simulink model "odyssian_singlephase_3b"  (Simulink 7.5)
settings: Solver=ode23t  StartTime=0.0  StopTime=10  RelTol=1e-6
undefined symbols (not defined in the file or in its folder): dfilt, DiscIntNeverNeededParam
libraries: powerlib x36, powerlib_extras x15, simulink x12, dsparch4 x2

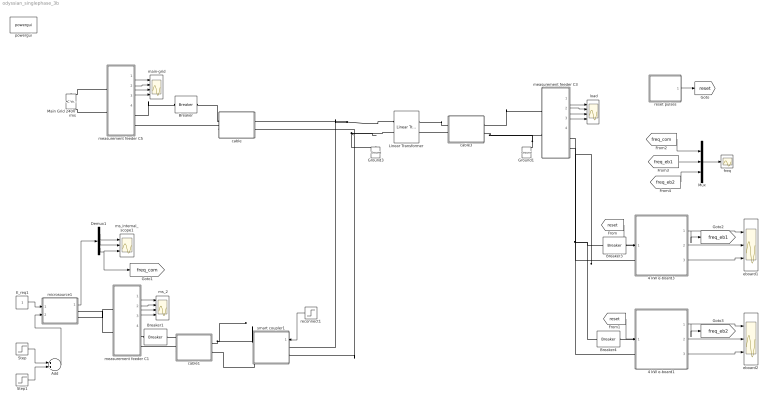
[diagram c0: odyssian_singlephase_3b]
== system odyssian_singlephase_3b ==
  " load" : Scope  NumInputPorts=4
  " main-grid" : Scope  NumInputPorts=4
  " ms_2" : Scope  NumInputPorts=4
  4 kW e-board1 : Subsystem  mask{tf=100, p=2}
      mask prompts: tf "fault_time"; p "load priority"
  4 kW e-board3 : Subsystem  mask{tf=100, p=1}
      mask prompts: tf "fault_time"; p "load priority"
  Add : Sum  OutDataType=fixdt(1, 16)  OutScaling=2^-10
  Breaker : powerlib/Elements/Breaker  DialogController=POWERSYS.PowerSysDialog  SystemSampleTime=-1  BreakerResistance=0.01  InitialState=1  SnubberResistance=1e6  SnubberCapacitance=inf  SwitchingTimes=[4]  External=off  Measurements=None  MoreParameters=off  NoBreakLoop=off
  Breaker1 : powerlib/Elements/Breaker  DialogController=POWERSYS.PowerSysDialog  SystemSampleTime=-1  BreakerResistance=0.01  InitialState=1  SnubberResistance=1e6  SnubberCapacitance=inf  SwitchingTimes=[100]  External=off  Measurements=None  MoreParameters=off  NoBreakLoop=off
  Breaker3 : powerlib/Elements/Breaker  DialogController=POWERSYS.PowerSysDialog  SystemSampleTime=-1  BreakerResistance=0.01  InitialState=1  SnubberResistance=1e6  SnubberCapacitance=inf  SwitchingTimes=[100]  External=off  Measurements=None  MoreParameters=off  NoBreakLoop=off
  Breaker4 : powerlib/Elements/Breaker  DialogController=POWERSYS.PowerSysDialog  SystemSampleTime=-1  BreakerResistance=0.01  InitialState=1  SnubberResistance=1e6  SnubberCapacitance=inf  SwitchingTimes=[100]  External=off  Measurements=None  MoreParameters=off  NoBreakLoop=off
  Demux1 : Demux  Outputs=3
  E_req1 : Constant  OutDataType=fixdt(1, 16)  OutScaling=2^0
  Ground1 : powerlib/Elements/Ground  DialogController=POWERSYS.PowerSysDialog  PhysicalDomain=powersysdomain  SubClassName=unknown  LeftPortType=p1  RightPortType=p1  LConnTagsString=a
  Ground3 : powerlib/Elements/Ground  DialogController=POWERSYS.PowerSysDialog  PhysicalDomain=powersysdomain  SubClassName=unknown  LeftPortType=p1  RightPortType=p1  LConnTagsString=a
  Linear Transformer : powerlib/Elements/Linear Transformer  DialogController=POWERSYS.PowerSysDialog  PhysicalDomain=powersysdomain  SubClassName=unknown  LeftPortType=p1  RightPortType=p1  LConnTagsString=a|b  RConnTagsString=A|B  UNITS=SI  NominalPower=[ 45e3 , 60 ]  winding1=[240 0.001 1.e-3]  winding2=[120 .001 1.e-3]  ThreeWindings=off  winding3=[3.15e+05 0.7938 0.084225]  RmLm=[1.0804e+06 2866]  Measurements=All voltages and currents  DataType=on
  Main Grid 240V rms : powerlib/Electrical Sources/AC Voltage Source  DialogController=POWERSYS.PowerSysDialog  SystemSampleTime=-1  Amplitude=240*sqrt(2)  Phase=0  Frequency=60  SampleTime=0  Measurements=None
  Mux : Mux  Inputs=3
  Step : Step  Time=3  Before=.8  After=.2  SampleTime=0
  Step1 : Step  Time=6  After=.6  SampleTime=0
  cable : Subsystem
  cable1 : Subsystem
  cable3 : Subsystem
  eboard1 : Scope  NumInputPorts=3
  eboard2 : Scope  NumInputPorts=3
  freq : Scope
  measurement feeder C1 : Subsystem
  measurement feeder C3 : Subsystem
  measurement feeder C5 : Subsystem
  microsource1 : Subsystem  AncestorBlock=|
      | UWM_blocks/inverter-based
      | DG (simplified)
      | 208V - 15kVA
  ms_internal_scope1 : Scope  NumInputPorts=3
  powergui : powerlib/powergui  Priority=1  SystemSampleTime=-1  SimulationMode=Discrete  SampleTime=50e-5  frequency=60  SPID=off  DisableSnubberDevices=off  DisableRonSwitches=off  DisableVfSwitches=off  SwTol=0  Interpol=off  frequencyindice=0  echomessages=off  HookPort=off  DisplayEquations=off  FunctionMessages=off  EnableUseOfTLC=off  x0status=blocks  RestoreLinks=warning  ResistiveCurrentMeasurement=off  Frange=[0:2:500]  Ylog=off  Xlog=on  ShowGrid=off  save=off  variable=ZData  ZoomFFT=on  StartTime=0.0  cycles=1  DisplayStyle=1  fundamental=60  FreqAxis=off  MaxFrequency=1000  frequencyindicesteady=1  RmsSteady=1  display=off  Ts=0  methode=off
  reconnect1 : Step  Time=.1  SampleTime=0
  reset pulses : Subsystem  mask{tpulse=[50 100]}
  smart coupler1 : Subsystem
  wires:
  measurement feeder C3/1(Vm) -> " load"/1
  measurement feeder C3/2(Im) -> " load"/2
  measurement feeder C3/3(PQ) -> " load"/3
  measurement feeder C3/4(RMS (V-I)) -> " load"/4
  4 kW e-board3/1(w) -> eboard1/1, [freq_eb1]
  4 kW e-board3/2(Irms) -> eboard1/2
  4 kW e-board3/3(Vrms) -> eboard1/3
  [reset] -> 4 kW e-board3/1(reset)
  4 kW e-board1/1(w) -> eboard2/1, [freq_eb2]
  4 kW e-board1/2(Irms) -> eboard2/2
  4 kW e-board1/3(Vrms) -> eboard2/3
  [reset] -> 4 kW e-board1/1(reset)
  Mux/1 -> freq/1
  reset pulses/1(Out1) -> [reset]
  [freq_com] -> Mux/1
  [freq_eb1] -> Mux/2
  [freq_eb2] -> Mux/3
  measurement feeder C5/1(Vm) -> " main-grid"/1
  measurement feeder C5/2(Im) -> " main-grid"/2
  measurement feeder C5/3(PQ) -> " main-grid"/3
  measurement feeder C5/4(RMS (V-I)) -> " main-grid"/4
  measurement feeder C1/1(Vm) -> " ms_2"/1
  measurement feeder C1/2(Im) -> " ms_2"/2
  measurement feeder C1/3(PQ) -> " ms_2"/3
  measurement feeder C1/4(RMS (V-I)) -> " ms_2"/4
  E_req1/1 -> microsource1/1(E_req)
  Demux1/2 -> ms_internal_scope1/2
  Demux1/1 -> ms_internal_scope1/1
  Demux1/3 -> ms_internal_scope1/3, [freq_com]
  microsource1/1(m) -> Demux1/1
  reconnect1/1 -> smart coupler1/1(switch)
  ? -> ?
  Step/1 -> Add/1
  Step1/1 -> Add/2
  Add/1 -> microsource1/2(P_req)
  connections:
  measurement feeder C3/RConn1 -- Breaker3/RConn1 -- Breaker4/RConn1
  measurement feeder C3/RConn2 -- 4 kW e-board3/LConn2 -- 4 kW e-board1/LConn2
  cable3/LConn2 -- Ground1/LConn1 -- measurement feeder C3/LConn2
  4 kW e-board3/LConn1 -- Breaker3/LConn1
  4 kW e-board1/LConn1 -- Breaker4/LConn1
  measurement feeder C5/RConn1 -- Breaker/LConn1
  cable/RConn2 -- measurement feeder C5/RConn2
  cable/RConn1 -- Breaker/RConn1
  Linear Transformer/LConn1 -- smart coupler1/LConn1 -- cable/LConn1
  Linear Transformer/LConn2 -- Ground3/LConn1 -- smart coupler1/LConn2 -- cable/LConn2
  cable3/LConn1 -- measurement feeder C3/LConn1
  cable3/RConn2 -- Linear Transformer/RConn2
  cable3/RConn1 -- Linear Transformer/RConn1
  measurement feeder C5/LConn1 -- Main Grid 240V rms/RConn1
  measurement feeder C5/LConn2 -- Main Grid 240V rms/LConn1
  smart coupler1/RConn2 -- cable1/LConn2
  cable1/LConn1 -- smart coupler1/RConn1
  cable1/RConn2 -- measurement feeder C1/RConn2
  measurement feeder C1/LConn1 -- microsource1/RConn1
  cable1/RConn1 -- Breaker1/LConn1
  measurement feeder C1/LConn2 -- microsource1/RConn2
  Breaker1/RConn1 -- measurement feeder C1/RConn1

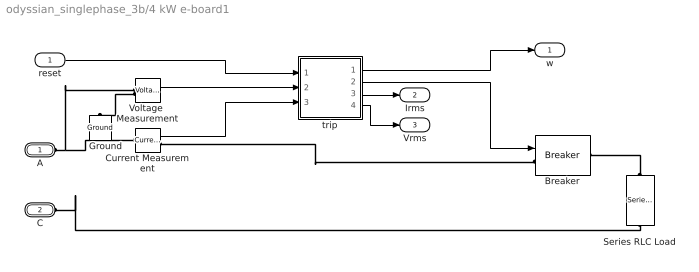
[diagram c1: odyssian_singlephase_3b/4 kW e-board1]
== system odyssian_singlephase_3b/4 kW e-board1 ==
  reset : Inport
  Breaker : powerlib/Elements/Breaker  DialogController=POWERSYS.PowerSysDialog  SystemSampleTime=-1  BreakerResistance=0.01  InitialState=1  SnubberResistance=1e6  SnubberCapacitance=inf  SwitchingTimes="[ 1/60  5/60 ]"  External=on  Measurements=None  MoreParameters=off  NoBreakLoop=off
  Current Measurement : powerlib/Measurements/Current Measurement  DialogController=POWERSYS.PowerSysDialog  SystemSampleTime=-1  PhasorSimulation=off  OutputType=Complex  PSBequivalent=0
  Ground : powerlib/Elements/Ground  DialogController=POWERSYS.PowerSysDialog  PhysicalDomain=powersysdomain  SubClassName=unknown  LeftPortType=p1  RightPortType=p1  LConnTagsString=a
  Series RLC Load : powerlib/Elements/Series RLC Load  DialogController=POWERSYS.PowerSysDialog  PhysicalDomain=powersysdomain  SubClassName=unknown  LeftPortType=p1  RightPortType=p1  LConnTagsString=a  RConnTagsString=__new0  NominalVoltage=120  NominalFrequency=60  ActivePower=60  InductivePower=0  CapacitivePower=0  Setx0=off  InitialVoltage=0  SetiL0=off  InitialCurrent=0  Measurements=None
  Voltage  Measurement : powerlib/Measurements/Voltage Measurement  DialogController=POWERSYS.PowerSysDialog  SystemSampleTime=-1  PhasorSimulation=off  OutputType=Complex  PSBequivalent=0
  trip : Subsystem  mask{p=p}
      mask prompts: p "priority level"
  A : PMIOPort  Port=1  Side=Left
  C : PMIOPort  Port=2  Side=Left
  w : Outport  OutDataType=fixdt(1, 16)  OutScaling=2^0
  Irms : Outport  Port=2  OutDataType=fixdt(1, 16)  OutScaling=2^0
  Vrms : Outport  Port=3  OutDataType=fixdt(1, 16)  OutScaling=2^0
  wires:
  trip/1(w) -> w/1
  Current Measurement/1 -> trip/3(I)
  Voltage  Measurement/1 -> trip/2(V)
  reset/1 -> trip/1(Reset)
  trip/2(trip) -> Breaker/1
  trip/3(Irms) -> Irms/1
  trip/4(Vrms) -> Vrms/1
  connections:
  A/RConn1 -- Current Measurement/LConn1 -- Voltage  Measurement/LConn1
  Voltage  Measurement/LConn2 -- Ground/LConn1
  Current Measurement/RConn1 -- Breaker/LConn1
  Series RLC Load/LConn1 -- Breaker/RConn1
  Series RLC Load/RConn1 -- C/RConn1

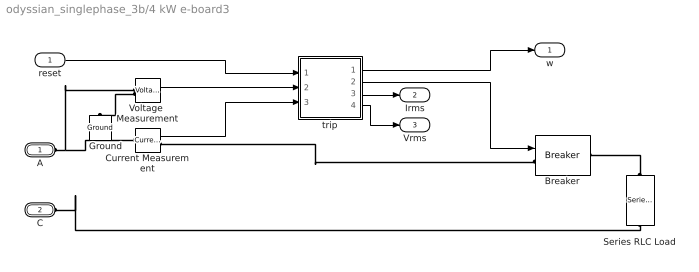
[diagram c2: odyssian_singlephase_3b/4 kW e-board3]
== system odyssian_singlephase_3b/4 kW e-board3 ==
  reset : Inport
  Breaker : powerlib/Elements/Breaker  DialogController=POWERSYS.PowerSysDialog  SystemSampleTime=-1  BreakerResistance=0.01  InitialState=1  SnubberResistance=1e6  SnubberCapacitance=inf  SwitchingTimes="[ 1/60  5/60 ]"  External=on  Measurements=None  MoreParameters=off  NoBreakLoop=off
  Current Measurement : powerlib/Measurements/Current Measurement  DialogController=POWERSYS.PowerSysDialog  SystemSampleTime=-1  PhasorSimulation=off  OutputType=Complex  PSBequivalent=0
  Ground : powerlib/Elements/Ground  DialogController=POWERSYS.PowerSysDialog  PhysicalDomain=powersysdomain  SubClassName=unknown  LeftPortType=p1  RightPortType=p1  LConnTagsString=a
  Series RLC Load : powerlib/Elements/Series RLC Load  DialogController=POWERSYS.PowerSysDialog  PhysicalDomain=powersysdomain  SubClassName=unknown  LeftPortType=p1  RightPortType=p1  LConnTagsString=a  RConnTagsString=__new0  NominalVoltage=120  NominalFrequency=60  ActivePower=120  InductivePower=0  CapacitivePower=0  Setx0=off  InitialVoltage=0  SetiL0=off  InitialCurrent=0  Measurements=None
  Voltage  Measurement : powerlib/Measurements/Voltage Measurement  DialogController=POWERSYS.PowerSysDialog  SystemSampleTime=-1  PhasorSimulation=off  OutputType=Complex  PSBequivalent=0
  trip : Subsystem  mask{p=p}
      mask prompts: p "priority level"
  A : PMIOPort  Port=1  Side=Left
  C : PMIOPort  Port=2  Side=Left
  w : Outport  OutDataType=fixdt(1, 16)  OutScaling=2^0
  Irms : Outport  Port=2  OutDataType=fixdt(1, 16)  OutScaling=2^0
  Vrms : Outport  Port=3  OutDataType=fixdt(1, 16)  OutScaling=2^0
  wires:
  trip/1(w) -> w/1
  Current Measurement/1 -> trip/3(I)
  Voltage  Measurement/1 -> trip/2(V)
  reset/1 -> trip/1(Reset)
  trip/2(trip) -> Breaker/1
  trip/3(Irms) -> Irms/1
  trip/4(Vrms) -> Vrms/1
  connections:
  A/RConn1 -- Current Measurement/LConn1 -- Voltage  Measurement/LConn1
  Voltage  Measurement/LConn2 -- Ground/LConn1
  Current Measurement/RConn1 -- Breaker/LConn1
  Series RLC Load/LConn1 -- Breaker/RConn1
  Series RLC Load/RConn1 -- C/RConn1

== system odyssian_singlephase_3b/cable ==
  Series RLC Branch : powerlib/Elements/Series RLC Branch  DialogController=POWERSYS.PowerSysDialog  PhysicalDomain=powersysdomain  SubClassName=unknown  LeftPortType=p1  RightPortType=p1  LConnTagsString=__new0  RConnTagsString=__new0  BranchType=RL  Resistance=.001  Inductance=1.e-5  SetiL0=off  InitialCurrent=0  Capacitance=1e-6  Setx0=off  InitialVoltage=0  Measurements=None
  A : PMIOPort  Tag=PMCPort  Port=1  Side=Left
  A' : PMIOPort  Tag=PMCPort  Port=2  Side=Right
  B' : PMIOPort  Tag=PMCPort  Port=3  Side=Right
  B : PMIOPort  Tag=PMCPort  Port=4  Side=Left
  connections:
  A/RConn1 -- Series RLC Branch/LConn1
  A'/RConn1 -- Series RLC Branch/RConn1
  B/RConn1 -- B'/RConn1

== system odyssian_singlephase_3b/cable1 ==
  Series RLC Branch : powerlib/Elements/Series RLC Branch  DialogController=POWERSYS.PowerSysDialog  PhysicalDomain=powersysdomain  SubClassName=unknown  LeftPortType=p1  RightPortType=p1  LConnTagsString=__new0  RConnTagsString=__new0  BranchType=RL  Resistance=.001  Inductance=1.e-6  SetiL0=off  InitialCurrent=0  Capacitance=1e-6  Setx0=off  InitialVoltage=0  Measurements=None
  A : PMIOPort  Tag=PMCPort  Port=1  Side=Left
  A' : PMIOPort  Tag=PMCPort  Port=2  Side=Right
  B' : PMIOPort  Tag=PMCPort  Port=3  Side=Right
  B : PMIOPort  Tag=PMCPort  Port=4  Side=Left
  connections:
  A/RConn1 -- Series RLC Branch/LConn1
  Series RLC Branch/RConn1 -- A'/RConn1
  B/RConn1 -- B'/RConn1

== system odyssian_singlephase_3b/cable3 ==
  Series RLC Branch : powerlib/Elements/Series RLC Branch  DialogController=POWERSYS.PowerSysDialog  PhysicalDomain=powersysdomain  SubClassName=unknown  LeftPortType=p1  RightPortType=p1  LConnTagsString=__new0  RConnTagsString=__new0  BranchType=RL  Resistance=.001  Inductance=1.e-6  SetiL0=off  InitialCurrent=0  Capacitance=1e-6  Setx0=off  InitialVoltage=0  Measurements=None
  A : PMIOPort  Tag=PMCPort  Port=1  Side=Left
  A' : PMIOPort  Tag=PMCPort  Port=2  Side=Right
  B' : PMIOPort  Tag=PMCPort  Port=3  Side=Right
  B : PMIOPort  Tag=PMCPort  Port=4  Side=Left
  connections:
  A/RConn1 -- Series RLC Branch/LConn1
  Series RLC Branch/RConn1 -- A'/RConn1
  B/RConn1 -- B'/RConn1

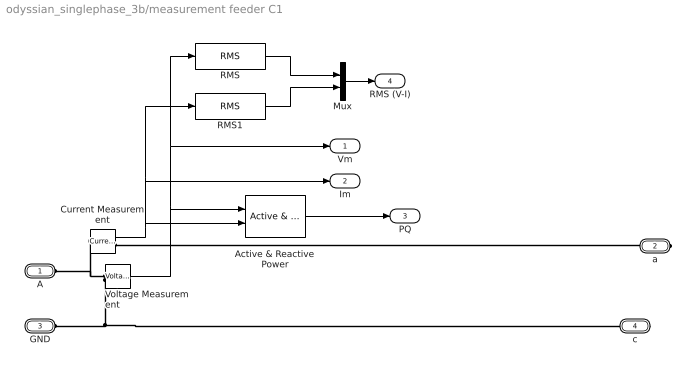
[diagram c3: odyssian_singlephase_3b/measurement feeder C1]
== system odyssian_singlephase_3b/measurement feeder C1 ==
  Active & Reactive Power : powerlib_extras/Measurements/Active & Reactive Power  DialogController=POWERSYS.PowerSysDialog  SystemSampleTime=-1  f1=60
  Current Measurement : powerlib/Measurements/Current Measurement  DialogController=POWERSYS.PowerSysDialog  SystemSampleTime=-1  PhasorSimulation=off  OutputType=Complex  PSBequivalent=0
  Mux : Mux  Inputs=2
  RMS : powerlib_extras/Measurements/RMS  DialogController=POWERSYS.PowerSysDialog  SystemSampleTime=-1  f1=60
  RMS1 : powerlib_extras/Measurements/RMS  DialogController=POWERSYS.PowerSysDialog  SystemSampleTime=-1  f1=60
  Voltage Measurement : powerlib/Measurements/Voltage Measurement  DialogController=POWERSYS.PowerSysDialog  SystemSampleTime=-1  PhasorSimulation=off  OutputType=Complex  PSBequivalent=0
  A : PMIOPort  Port=1  Side=Left
  a : PMIOPort  Port=2  Side=Right
  GND : PMIOPort  Port=3  Side=Left
  c : PMIOPort  Port=4  Side=Right
  Vm : Outport  OutDataType=fixdt(1, 16)  OutScaling=2^0
  Im : Outport  Port=2  OutDataType=fixdt(1, 16)  OutScaling=2^0
  PQ : Outport  Port=3  OutDataType=fixdt(1, 16)  OutScaling=2^0
  RMS (V-I) : Outport  Port=4  OutDataType=fixdt(1, 16)  OutScaling=2^0
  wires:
  Mux/1 -> RMS (V-I)/1
  Current Measurement/1 -> Im/1, RMS1/1, Active & Reactive Power/2
  Voltage Measurement/1 -> Vm/1, RMS/1, Active & Reactive Power/1
  Active & Reactive Power/1 -> PQ/1
  RMS/1 -> Mux/1
  RMS1/1 -> Mux/2
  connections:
  a/RConn1 -- Current Measurement/RConn1
  Voltage Measurement/LConn1 -- A/RConn1 -- Current Measurement/LConn1
  Voltage Measurement/LConn2 -- GND/RConn1 -- c/RConn1

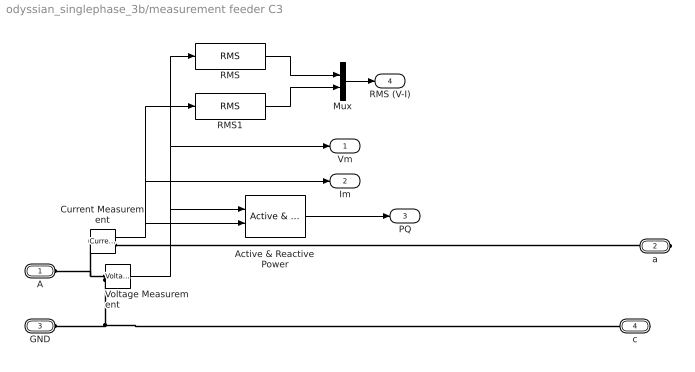
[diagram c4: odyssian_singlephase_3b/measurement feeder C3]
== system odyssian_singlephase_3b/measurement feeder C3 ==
  Active & Reactive Power : powerlib_extras/Measurements/Active & Reactive Power  DialogController=POWERSYS.PowerSysDialog  SystemSampleTime=-1  f1=60
  Current Measurement : powerlib/Measurements/Current Measurement  DialogController=POWERSYS.PowerSysDialog  SystemSampleTime=-1  PhasorSimulation=off  OutputType=Complex  PSBequivalent=0
  Mux : Mux  Inputs=2
  RMS : powerlib_extras/Measurements/RMS  DialogController=POWERSYS.PowerSysDialog  SystemSampleTime=-1  f1=60
  RMS1 : powerlib_extras/Measurements/RMS  DialogController=POWERSYS.PowerSysDialog  SystemSampleTime=-1  f1=60
  Voltage Measurement : powerlib/Measurements/Voltage Measurement  DialogController=POWERSYS.PowerSysDialog  SystemSampleTime=-1  PhasorSimulation=off  OutputType=Complex  PSBequivalent=0
  A : PMIOPort  Port=1  Side=Left
  a : PMIOPort  Port=2  Side=Right
  GND : PMIOPort  Port=3  Side=Left
  c : PMIOPort  Port=4  Side=Right
  Vm : Outport  OutDataType=fixdt(1, 16)  OutScaling=2^0
  Im : Outport  Port=2  OutDataType=fixdt(1, 16)  OutScaling=2^0
  PQ : Outport  Port=3  OutDataType=fixdt(1, 16)  OutScaling=2^0
  RMS (V-I) : Outport  Port=4  OutDataType=fixdt(1, 16)  OutScaling=2^0
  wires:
  Mux/1 -> RMS (V-I)/1
  Current Measurement/1 -> Im/1, RMS1/1, Active & Reactive Power/2
  Voltage Measurement/1 -> Vm/1, RMS/1, Active & Reactive Power/1
  Active & Reactive Power/1 -> PQ/1
  RMS/1 -> Mux/1
  RMS1/1 -> Mux/2
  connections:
  a/RConn1 -- Current Measurement/RConn1
  Voltage Measurement/LConn1 -- A/RConn1 -- Current Measurement/LConn1
  Voltage Measurement/LConn2 -- GND/RConn1 -- c/RConn1

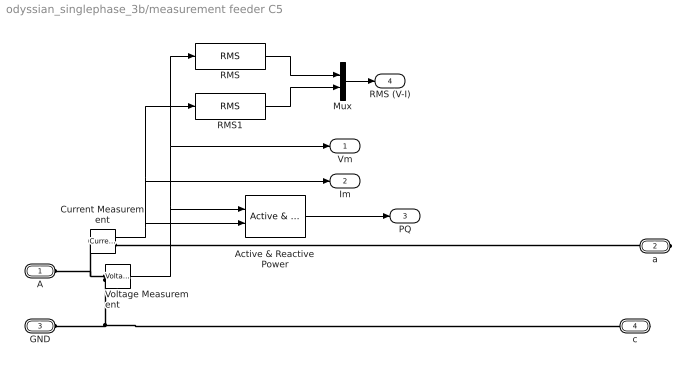
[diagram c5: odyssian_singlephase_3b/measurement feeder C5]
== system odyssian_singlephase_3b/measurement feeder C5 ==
  Active & Reactive Power : powerlib_extras/Measurements/Active & Reactive Power  DialogController=POWERSYS.PowerSysDialog  SystemSampleTime=-1  f1=60
  Current Measurement : powerlib/Measurements/Current Measurement  DialogController=POWERSYS.PowerSysDialog  SystemSampleTime=-1  PhasorSimulation=off  OutputType=Complex  PSBequivalent=0
  Mux : Mux  Inputs=2
  RMS : powerlib_extras/Measurements/RMS  DialogController=POWERSYS.PowerSysDialog  SystemSampleTime=-1  f1=60
  RMS1 : powerlib_extras/Measurements/RMS  DialogController=POWERSYS.PowerSysDialog  SystemSampleTime=-1  f1=60
  Voltage Measurement : powerlib/Measurements/Voltage Measurement  DialogController=POWERSYS.PowerSysDialog  SystemSampleTime=-1  PhasorSimulation=off  OutputType=Complex  PSBequivalent=0
  A : PMIOPort  Port=1  Side=Left
  a : PMIOPort  Port=2  Side=Right
  GND : PMIOPort  Port=3  Side=Left
  c : PMIOPort  Port=4  Side=Right
  Vm : Outport  OutDataType=fixdt(1, 16)  OutScaling=2^0
  Im : Outport  Port=2  OutDataType=fixdt(1, 16)  OutScaling=2^0
  PQ : Outport  Port=3  OutDataType=fixdt(1, 16)  OutScaling=2^0
  RMS (V-I) : Outport  Port=4  OutDataType=fixdt(1, 16)  OutScaling=2^0
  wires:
  Mux/1 -> RMS (V-I)/1
  Current Measurement/1 -> Im/1, RMS1/1, Active & Reactive Power/2
  Voltage Measurement/1 -> Vm/1, RMS/1, Active & Reactive Power/1
  Active & Reactive Power/1 -> PQ/1
  RMS/1 -> Mux/1
  RMS1/1 -> Mux/2
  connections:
  a/RConn1 -- Current Measurement/RConn1
  Voltage Measurement/LConn1 -- A/RConn1 -- Current Measurement/LConn1
  Voltage Measurement/LConn2 -- GND/RConn1 -- c/RConn1

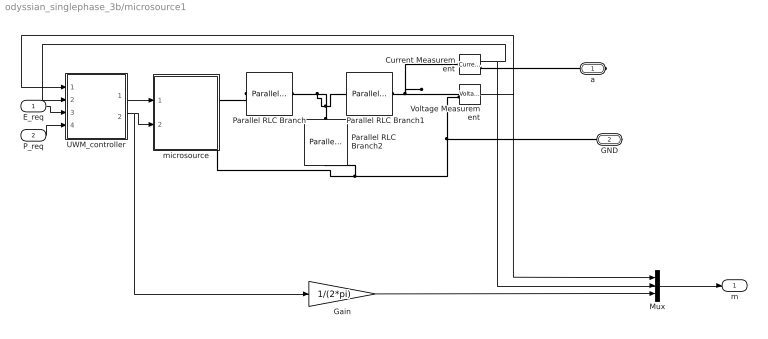
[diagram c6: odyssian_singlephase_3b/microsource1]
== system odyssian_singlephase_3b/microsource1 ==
  E_req : Inport
  P_req : Inport  Port=2
  Current Measurement : powerlib/Measurements/Current Measurement  DialogController=POWERSYS.PowerSysDialog  SystemSampleTime=-1  PhasorSimulation=off  OutputType=Complex  PSBequivalent=0
  Gain : Gain  Gain=1/(2*pi)  ParameterDataType=fixdt(1, 16)  ParameterScaling=2^0  OutDataType=fixdt(1, 16)  OutScaling=2^0
  Mux : Mux  Inputs=3
  Parallel RLC Branch : powerlib/Elements/Parallel RLC Branch  DialogController=POWERSYS.PowerSysDialog  PhysicalDomain=powersysdomain  SubClassName=unknown  LeftPortType=p1  RightPortType=p1  LConnTagsString=a  RConnTagsString=__new0  BranchType=L  Resistance=1  Inductance=1.e-1  SetiL0=off  InitialCurrent=0  Capacitance=1e-6  Setx0=off  InitialVoltage=0  Measurements=None
  Parallel RLC Branch1 : powerlib/Elements/Parallel RLC Branch  DialogController=POWERSYS.PowerSysDialog  PhysicalDomain=powersysdomain  SubClassName=unknown  LeftPortType=p1  RightPortType=p1  LConnTagsString=a  RConnTagsString=__new0  BranchType=L  Resistance=1  Inductance=1.e-1  SetiL0=off  InitialCurrent=0  Capacitance=1e-6  Setx0=off  InitialVoltage=0  Measurements=None
  Parallel RLC Branch2 : powerlib/Elements/Parallel RLC Branch  DialogController=POWERSYS.PowerSysDialog  PhysicalDomain=powersysdomain  SubClassName=unknown  LeftPortType=p1  RightPortType=p1  LConnTagsString=a  RConnTagsString=__new0  BranchType=C  Resistance=1  Inductance=1.e-1  SetiL0=off  InitialCurrent=0  Capacitance=1.e-5  Setx0=off  InitialVoltage=0  Measurements=None
  UWM_controller : Subsystem  mask{Vbase=240*sqrt(2), Sbase=200}
  Voltage Measurement : powerlib/Measurements/Voltage Measurement  DialogController=POWERSYS.PowerSysDialog  SystemSampleTime=-1  PhasorSimulation=off  OutputType=Complex  PSBequivalent=0
  microsource : Subsystem
  a : PMIOPort  Port=1  Side=Right
  GND : PMIOPort  Port=2  Side=Right
  m : Outport  OutDataType=fixdt(1, 16)  OutScaling=2^0
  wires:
  E_req/1 -> UWM_controller/3(E_req)
  P_req/1 -> UWM_controller/4(P_req)
  UWM_controller/1(Vpk) -> microsource/1(Vpk)
  UWM_controller/2(w) -> microsource/2(w), Gain/1
  Mux/1 -> m/1
  Gain/1 -> Mux/3
  Current Measurement/1 -> Mux/2, UWM_controller/2(i_meas)
  Voltage Measurement/1 -> Mux/1, UWM_controller/1(v_meas)
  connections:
  Voltage Measurement/LConn2 -- GND/RConn1 -- Parallel RLC Branch2/RConn1 -- microsource/RConn2
  Parallel RLC Branch1/RConn1 -- Voltage Measurement/LConn1 -- Current Measurement/LConn1
  a/RConn1 -- Current Measurement/RConn1
  Parallel RLC Branch/LConn1 -- microsource/RConn1
  Parallel RLC Branch2/LConn1 -- Parallel RLC Branch1/LConn1 -- Parallel RLC Branch/RConn1

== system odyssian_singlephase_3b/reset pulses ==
  Sum : Sum  Inputs=|++  OutDataType=fixdt(1, 16)  OutScaling=2^0
  pulse : Subsystem  mask{tstart=tpulse(1), dt=.1}
  pulse1 : Subsystem  mask{tstart=tpulse(2), dt=.1}
  Out1 : Outport
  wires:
  pulse/1(Out1) -> Sum/1
  pulse1/1(Out1) -> Sum/2
  Sum/1 -> Out1/1

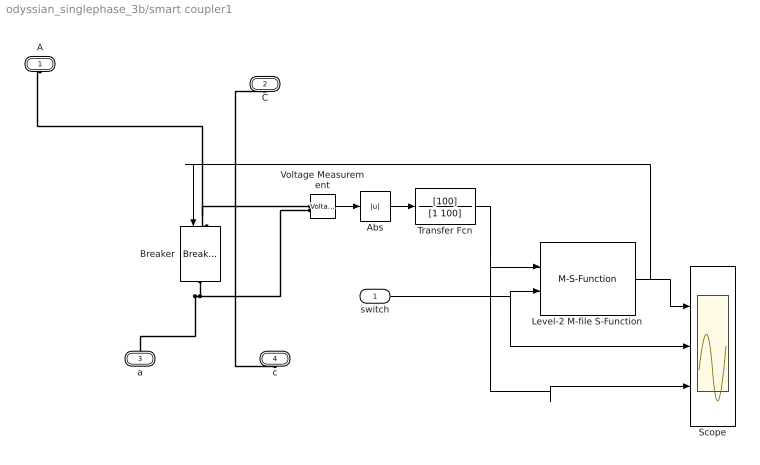
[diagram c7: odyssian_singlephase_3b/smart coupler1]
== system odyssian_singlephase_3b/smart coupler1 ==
  switch : Inport  OutDataType=fixdt(1, 16)  OutScaling=2^0
  Abs : Abs  OutDataType=fixdt(1, 16)  OutScaling=2^0
  Breaker : powerlib/Elements/Breaker  DialogController=POWERSYS.PowerSysDialog  SystemSampleTime=-1  BreakerResistance=0.01  InitialState=0  SnubberResistance=1e6  SnubberCapacitance=inf  SwitchingTimes="[ 1/60  5/60 ]"  External=on  Measurements=None  MoreParameters=off  NoBreakLoop=off
  Level-2 M-file S-Function : M-S-Function  FunctionName=smart_coupler
  Scope : Scope  NumInputPorts=3
  Transfer Fcn : TransferFcn  Numerator=[100]  Denominator=[1 100]
  Voltage Measurement : powerlib/Measurements/Voltage Measurement  DialogController=POWERSYS.PowerSysDialog  SystemSampleTime=-1  PhasorSimulation=off  OutputType=Complex  PSBequivalent=0
  A : PMIOPort  Port=1  Side=Left
  C : PMIOPort  Port=2  Side=Left
  a : PMIOPort  Port=3  Side=Right
  c : PMIOPort  Port=4  Side=Right
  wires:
  switch/1 -> Level-2 M-file S-Function/2, Scope/2
  Level-2 M-file S-Function/1 -> Scope/1, Breaker/1
  Voltage Measurement/1 -> Abs/1
  Abs/1 -> Transfer Fcn/1
  Transfer Fcn/1 -> Level-2 M-file S-Function/1, Scope/3
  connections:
  Breaker/LConn1 -- A/RConn1 -- Voltage Measurement/LConn1
  Breaker/RConn1 -- Voltage Measurement/LConn2 -- a/RConn1
  c/RConn1 -- C/RConn1

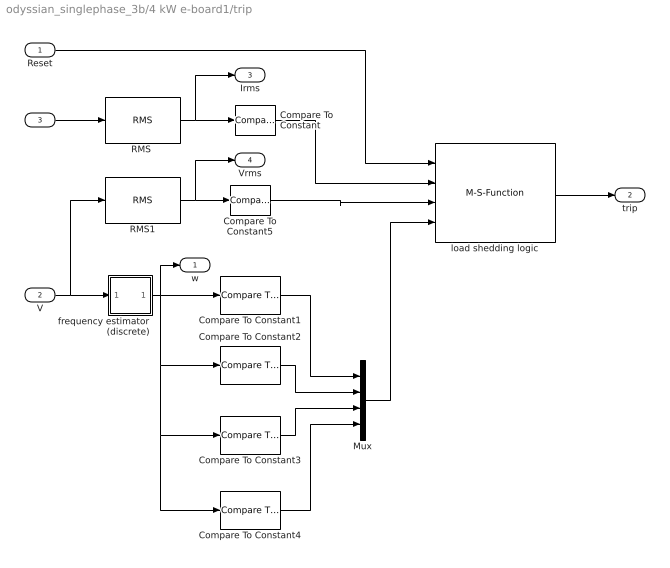
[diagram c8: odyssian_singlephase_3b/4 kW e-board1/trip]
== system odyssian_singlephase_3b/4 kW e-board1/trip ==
  Reset : Inport
  V : Inport  Port=2
  I : Inport  Port=3
  Compare To Constant : simulink/Logic and Bit Operations/Compare To Constant  SystemSampleTime=-1  relop=>=  const=100  LogicOutDataTypeMode=boolean
  Compare To Constant1 : simulink/Logic and Bit Operations/Compare To Constant  SystemSampleTime=-1  relop=<=  const=59.8  LogicOutDataTypeMode=boolean
  Compare To Constant2 : simulink/Logic and Bit Operations/Compare To Constant  SystemSampleTime=-1  relop=<=  const=59.5  LogicOutDataTypeMode=boolean
  Compare To Constant3 : simulink/Logic and Bit Operations/Compare To Constant  SystemSampleTime=-1  relop=>=  const=60.1  LogicOutDataTypeMode=boolean
  Compare To Constant4 : simulink/Logic and Bit Operations/Compare To Constant  SystemSampleTime=-1  relop=<=  const=58.6  LogicOutDataTypeMode=boolean
  Compare To Constant5 : simulink/Logic and Bit Operations/Compare To Constant  SystemSampleTime=-1  relop=<=  const=100  LogicOutDataTypeMode=boolean
  Mux : Mux
  "RMS " : powerlib_extras/Measurements/RMS  DialogController=POWERSYS.PowerSysDialog  SystemSampleTime=-1  f1=60
  RMS1 : powerlib_extras/Measurements/RMS  DialogController=POWERSYS.PowerSysDialog  SystemSampleTime=-1  f1=60
  frequency estimator (discrete) : Subsystem  mask{dt=0.010}
      mask prompts: dt "sample time"
  load shedding logic : M-S-Function  FunctionName=load_shedding_logic  Parameters=p
  w : Outport  OutDataType=fixdt(1, 16)  OutScaling=2^0
  trip : Outport  Port=2
  Irms : Outport  Port=3  OutDataType=fixdt(1, 16)  OutScaling=2^0
  Vrms : Outport  Port=4  OutDataType=fixdt(1, 16)  OutScaling=2^0
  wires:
  "RMS "/1 -> Compare To Constant/1, Irms/1
  I/1 -> "RMS "/1
  Reset/1 -> load shedding logic/1
  Compare To Constant/1 -> load shedding logic/2
  load shedding logic/1 -> trip/1
  V/1 -> frequency estimator (discrete)/1(v), RMS1/1
  frequency estimator (discrete)/1(w) -> Compare To Constant1/1, w/1, Compare To Constant2/1, Compare To Constant3/1, Compare To Constant4/1
  Compare To Constant1/1 -> Mux/1
  Compare To Constant2/1 -> Mux/2
  Compare To Constant3/1 -> Mux/3
  Compare To Constant4/1 -> Mux/4
  RMS1/1 -> Compare To Constant5/1, Vrms/1
  Compare To Constant5/1 -> load shedding logic/3
  Mux/1 -> load shedding logic/4

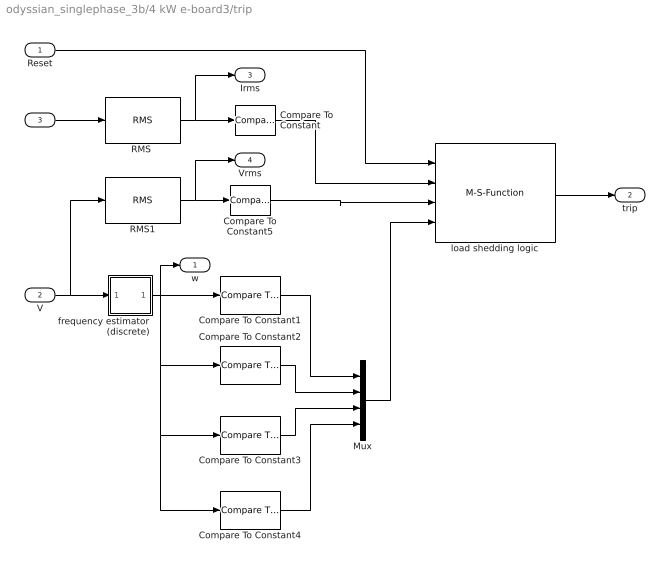
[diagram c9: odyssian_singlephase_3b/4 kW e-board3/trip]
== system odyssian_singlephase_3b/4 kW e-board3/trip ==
  Reset : Inport
  V : Inport  Port=2
  I : Inport  Port=3
  Compare To Constant : simulink/Logic and Bit Operations/Compare To Constant  SystemSampleTime=-1  relop=>=  const=100  LogicOutDataTypeMode=boolean
  Compare To Constant1 : simulink/Logic and Bit Operations/Compare To Constant  SystemSampleTime=-1  relop=<=  const=59.8  LogicOutDataTypeMode=boolean
  Compare To Constant2 : simulink/Logic and Bit Operations/Compare To Constant  SystemSampleTime=-1  relop=<=  const=59.5  LogicOutDataTypeMode=boolean
  Compare To Constant3 : simulink/Logic and Bit Operations/Compare To Constant  SystemSampleTime=-1  relop=>=  const=60.1  LogicOutDataTypeMode=boolean
  Compare To Constant4 : simulink/Logic and Bit Operations/Compare To Constant  SystemSampleTime=-1  relop=<=  const=58.6  LogicOutDataTypeMode=boolean
  Compare To Constant5 : simulink/Logic and Bit Operations/Compare To Constant  SystemSampleTime=-1  relop=<=  const=100  LogicOutDataTypeMode=boolean
  Mux : Mux
  "RMS " : powerlib_extras/Measurements/RMS  DialogController=POWERSYS.PowerSysDialog  SystemSampleTime=-1  f1=60
  RMS1 : powerlib_extras/Measurements/RMS  DialogController=POWERSYS.PowerSysDialog  SystemSampleTime=-1  f1=60
  frequency estimator (discrete) : Subsystem  mask{dt=0.010}
      mask prompts: dt "sample time"
  load shedding logic : M-S-Function  FunctionName=load_shedding_logic  Parameters=p
  w : Outport  OutDataType=fixdt(1, 16)  OutScaling=2^0
  trip : Outport  Port=2
  Irms : Outport  Port=3  OutDataType=fixdt(1, 16)  OutScaling=2^0
  Vrms : Outport  Port=4  OutDataType=fixdt(1, 16)  OutScaling=2^0
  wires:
  "RMS "/1 -> Compare To Constant/1, Irms/1
  I/1 -> "RMS "/1
  Reset/1 -> load shedding logic/1
  Compare To Constant/1 -> load shedding logic/2
  load shedding logic/1 -> trip/1
  V/1 -> frequency estimator (discrete)/1(v), RMS1/1
  frequency estimator (discrete)/1(w) -> Compare To Constant1/1, w/1, Compare To Constant2/1, Compare To Constant3/1, Compare To Constant4/1
  Compare To Constant1/1 -> Mux/1
  Compare To Constant2/1 -> Mux/2
  Compare To Constant3/1 -> Mux/3
  Compare To Constant4/1 -> Mux/4
  RMS1/1 -> Compare To Constant5/1, Vrms/1
  Compare To Constant5/1 -> load shedding logic/3
  Mux/1 -> load shedding logic/4

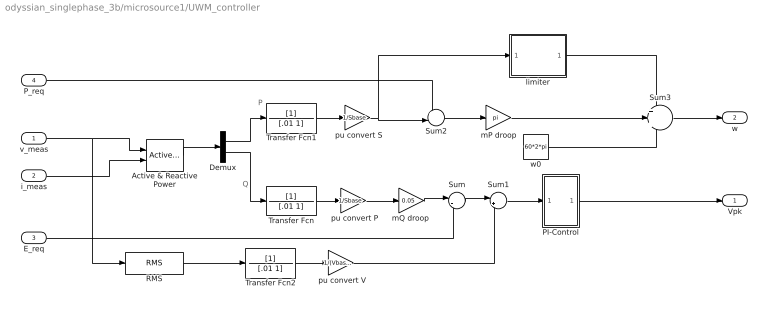
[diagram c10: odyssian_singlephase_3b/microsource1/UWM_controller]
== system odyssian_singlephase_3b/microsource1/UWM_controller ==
  note: P
  note: Q
  v_meas : Inport
  i_meas : Inport  Port=2
  E_req : Inport  Port=3
  P_req : Inport  Port=4
  " pu convert P" : Gain  Gain=1/Sbase  ParameterDataType=sfix(16)  ParameterScaling=2^0  OutDataType=sfix(16)  OutScaling=2^0
  " pu convert S" : Gain  Gain=1/Sbase  ParameterDataType=sfix(16)  ParameterScaling=2^0  OutDataType=sfix(16)  OutScaling=2^0
  " pu convert V" : Gain  Gain=1/(Vbase/sqrt(2))  ParameterDataType=sfix(16)  ParameterScaling=2^0  OutDataType=sfix(16)  OutScaling=2^0
  Active & Reactive Power : powerlib_extras/Measurements/Active & Reactive Power  DialogController=POWERSYS.PowerSysDialog  SystemSampleTime=-1  f1=60
  Demux : Demux  Outputs=2
  PI-Control : Subsystem
  RMS : powerlib_extras/Measurements/RMS  DialogController=POWERSYS.PowerSysDialog  SystemSampleTime=-1  f1=60
  Sum : Sum  Inputs=|-+  OutDataType=sfix(16)  OutScaling=2^0
  Sum1 : Sum  Inputs=|+-  OutDataType=sfix(16)  OutScaling=2^0
  Sum2 : Sum  Inputs=+-|  OutDataType=sfix(16)  OutScaling=2^0
  Sum3 : Sum  Inputs=+++  OutDataType=sfix(16)  OutScaling=2^0
  Transfer Fcn : TransferFcn  Denominator=[.01 1]
  Transfer Fcn1 : TransferFcn  Denominator=[.01 1]
  Transfer Fcn2 : TransferFcn  Denominator=[.01 1]
  limiter : Subsystem
  mP droop : Gain  Gain=pi  ParameterDataType=sfix(16)  ParameterScaling=2^0  OutDataType=sfix(16)  OutScaling=2^0
  "mQ droop " : Gain  Gain=0.05  ParameterDataType=sfix(16)  ParameterScaling=2^0  OutDataType=sfix(16)  OutScaling=2^0
  w0 : Constant  Value=60*2*pi  OutDataType=fixdt(1, 16)  OutScaling=2^0
  Vpk : Outport
  w : Outport  Port=2
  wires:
  Transfer Fcn2/1 -> " pu convert V"/1
  Transfer Fcn/1 -> " pu convert P"/1
  " pu convert P"/1 -> "mQ droop "/1
  Transfer Fcn1/1 -> " pu convert S"/1
  " pu convert S"/1 -> limiter/1(In1), Sum2/2
  i_meas/1 -> Active & Reactive Power/2
  P_req/1 -> Sum2/1
  mP droop/1 -> Sum3/2
  limiter/1(Out1) -> Sum3/1
  w0/1 -> Sum3/3
  Sum2/1 -> mP droop/1
  Sum1/1 -> PI-Control/1(In1)
  Sum/1 -> Sum1/1
  "mQ droop "/1 -> Sum/1
  Demux/2 -> Transfer Fcn/1
  Demux/1 -> Transfer Fcn1/1
  Active & Reactive Power/1 -> Demux/1
  v_meas/1 -> RMS/1, Active & Reactive Power/1
  PI-Control/1(Out1) -> Vpk/1
  Sum3/1 -> w/1
  E_req/1 -> Sum/2
  " pu convert V"/1 -> Sum1/2
  RMS/1 -> Transfer Fcn2/1

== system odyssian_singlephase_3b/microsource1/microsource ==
  Vpk : Inport  OutDataType=fixdt(1, 16)  OutScaling=2^0
  w : Inport  Port=2  OutDataType=fixdt(1, 16)  OutScaling=2^0
  Integrator : Integrator
  Product : Product  OutDataType=sfix(16)  OutScaling=2^0
  phaseA : powerlib/Electrical Sources/Controlled Voltage Source  DialogController=POWERSYS.PowerSysDialog  SystemSampleTime=-1  Initialize=on  Source_Type=AC  Amplitude=0  Phase=0  Frequency=0  Measurements=None
  v_A : Fcn  Expr=cos(u)
  Va : PMIOPort  Tag=PMCPort  Port=1  Side=Right
  Neutral : PMIOPort  Tag=PMCPort  Port=2  Side=Right
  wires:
  Product/1 -> phaseA/1
  Vpk/1 -> Product/1
  w/1 -> Integrator/1
  Integrator/1 -> v_A/1
  v_A/1 -> Product/2
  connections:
  phaseA/RConn1 -- Va/RConn1
  phaseA/LConn1 -- Neutral/RConn1

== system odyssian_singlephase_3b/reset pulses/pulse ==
  Step : Step  Time=tstart  SampleTime=0
  Step1 : Step  Time=tstart+dt  After=-1  SampleTime=0
  Sum : Sum  Inputs=|++  OutDataType=fixdt(1, 16)  OutScaling=2^0
  Out1 : Outport
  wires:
  Step/1 -> Sum/2
  Step1/1 -> Sum/1
  Sum/1 -> Out1/1

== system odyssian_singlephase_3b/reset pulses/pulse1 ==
  Step : Step  Time=tstart  SampleTime=0
  Step1 : Step  Time=tstart+dt  After=-1  SampleTime=0
  Sum : Sum  Inputs=|++  OutDataType=fixdt(1, 16)  OutScaling=2^0
  Out1 : Outport
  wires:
  Step/1 -> Sum/2
  Step1/1 -> Sum/1
  Sum/1 -> Out1/1

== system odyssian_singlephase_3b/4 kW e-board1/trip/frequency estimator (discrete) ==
  v : Inport
  Constant : Constant  Value=60  OutDataType=fixdt(1, 16)  OutScaling=2^0
  Fcn : Fcn  Expr=sin(2*pi*u[1])
  Filter Quantized : Subsystem  Tag=BlockMethodSubSystem
  Gain : Gain  Gain=1/150  ParameterDataType=fixdt(1, 16)  ParameterScaling=2^0  OutDataType=fixdt(1, 16)  OutScaling=2^0  SampleTime=dt
  Product : Product  OutDataType=fixdt(1, 16)  OutScaling=2^0
  Scope : Scope
  Sum : Sum  Inputs=|++  OutDataType=fixdt(1, 16)  OutScaling=2^0
  modulo discrete integrator : Subsystem  mask{dt=dt}
      mask prompts: dt "sample time"
  w : Outport  OutDataType=fixdt(1, 16)  OutScaling=2^0
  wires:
  Fcn/1 -> Product/2
  Constant/1 -> Sum/2
  modulo discrete integrator/1(Out1) -> Fcn/1
  Sum/1 -> modulo discrete integrator/1(In1), w/1
  Product/1 -> Filter Quantized/1(In)
  Filter Quantized/1(Out) -> Scope/1, Sum/1
  v/1 -> Gain/1
  Gain/1 -> Product/1

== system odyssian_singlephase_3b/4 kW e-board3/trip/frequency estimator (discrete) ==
  v : Inport
  Constant : Constant  Value=60  OutDataType=fixdt(1, 16)  OutScaling=2^0
  Fcn : Fcn  Expr=sin(2*pi*u[1])
  Filter Quantized : Subsystem  Tag=BlockMethodSubSystem
  Gain : Gain  Gain=1/150  ParameterDataType=fixdt(1, 16)  ParameterScaling=2^0  OutDataType=fixdt(1, 16)  OutScaling=2^0  SampleTime=dt
  Product : Product  OutDataType=fixdt(1, 16)  OutScaling=2^0
  Scope : Scope
  Sum : Sum  Inputs=|++  OutDataType=fixdt(1, 16)  OutScaling=2^0
  modulo discrete integrator : Subsystem  mask{dt=dt}
      mask prompts: dt "sample time"
  w : Outport  OutDataType=fixdt(1, 16)  OutScaling=2^0
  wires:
  Fcn/1 -> Product/2
  Constant/1 -> Sum/2
  modulo discrete integrator/1(Out1) -> Fcn/1
  Sum/1 -> modulo discrete integrator/1(In1), w/1
  Product/1 -> Filter Quantized/1(In)
  Filter Quantized/1(Out) -> Scope/1, Sum/1
  v/1 -> Gain/1
  Gain/1 -> Product/1

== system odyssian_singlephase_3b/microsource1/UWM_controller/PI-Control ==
  In1 : Inport
  Gain : Gain  Gain=.01  ParameterDataType=sfix(16)  ParameterScaling=2^0  OutDataType=sfix(16)  OutScaling=2^0
  Gain1 : Gain  Gain=5  ParameterDataType=sfix(16)  ParameterScaling=2^0  OutDataType=sfix(16)  OutScaling=2^0
  Gain2 : Gain  Gain=750  ParameterDataType=sfix(16)  ParameterScaling=2^0  OutDataType=sfix(16)  OutScaling=2^0
  Integrator1 : Integrator  LimitOutput=on  UpperSaturationLimit=100  LowerSaturationLimit=-100  ZeroCross=off
  Sum4 : Sum  Inputs=|++  OutDataType=sfix(16)  OutScaling=2^0
  Out1 : Outport
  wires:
  Gain/1 -> Sum4/1
  Integrator1/1 -> Sum4/2
  In1/1 -> Gain1/1, Gain/1
  Gain1/1 -> Integrator1/1
  Sum4/1 -> Gain2/1
  Gain2/1 -> Out1/1

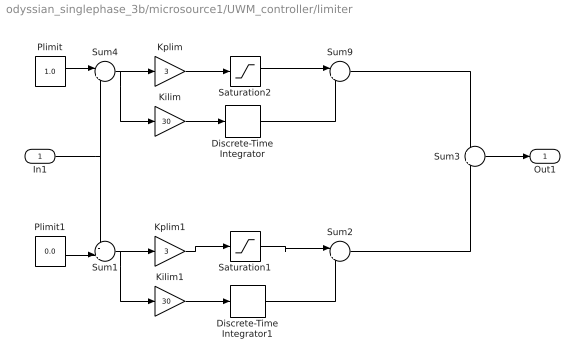
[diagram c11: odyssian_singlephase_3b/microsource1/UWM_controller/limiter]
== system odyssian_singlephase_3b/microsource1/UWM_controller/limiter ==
  In1 : Inport
  Discrete-Time Integrator : DiscreteIntegrator  OutDataType=fixdt(1, 16)  OutScaling=2^0  LimitOutput=on  UpperSaturationLimit=0  LowerSaturationLimit=-pi  ICPrevOutput=DiscIntNeverNeededParam  ICPrevScaledInput=DiscIntNeverNeededParam
  Discrete-Time Integrator1 : DiscreteIntegrator  OutDataType=fixdt(1, 16)  OutScaling=2^0  LimitOutput=on  UpperSaturationLimit=pi  LowerSaturationLimit=0  ICPrevOutput=DiscIntNeverNeededParam  ICPrevScaledInput=DiscIntNeverNeededParam
  Kilim : Gain  Gain=30  ParameterDataType=sfix(16)  ParameterScaling=2^0  OutDataType=sfix(16)  OutScaling=2^0
  Kilim1 : Gain  Gain=30  ParameterDataType=sfix(16)  ParameterScaling=2^0  OutDataType=sfix(16)  OutScaling=2^0
  Kplim : Gain  Gain=3  ParameterDataType=sfix(16)  ParameterScaling=2^0  OutDataType=sfix(16)  OutScaling=2^0
  Kplim1 : Gain  Gain=3  ParameterDataType=sfix(16)  ParameterScaling=2^0  OutDataType=sfix(16)  OutScaling=2^0
  Plimit : Constant  Value=1.0  OutDataType=sfix(16)  OutScaling=2^0
  Plimit1 : Constant  Value=0.0  OutDataType=sfix(16)  OutScaling=2^0
  Saturation1 : Saturate  UpperLimit=pi  LowerLimit=0  OutDataType=fixdt(1, 16)  OutScaling=2^0
  Saturation2 : Saturate  UpperLimit=0  LowerLimit=-pi  OutDataType=fixdt(1, 16)  OutScaling=2^0
  Sum1 : Sum  Inputs=-+|  OutDataType=sfix(16)  OutScaling=2^0
  Sum2 : Sum  Inputs=|++  OutDataType=sfix(16)  OutScaling=2^0
  Sum3 : Sum  OutDataType=sfix(16)  OutScaling=2^0
  Sum4 : Sum  Inputs=|+-  OutDataType=sfix(16)  OutScaling=2^0
  Sum9 : Sum  Inputs=|++  OutDataType=sfix(16)  OutScaling=2^0
  Out1 : Outport
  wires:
  Sum3/1 -> Out1/1
  Plimit1/1 -> Sum1/2
  Discrete-Time Integrator1/1 -> Sum2/2
  Kilim1/1 -> Discrete-Time Integrator1/1
  Sum1/1 -> Kilim1/1, Kplim1/1
  In1/1 -> Sum1/1, Sum4/2
  Discrete-Time Integrator/1 -> Sum9/2
  Kilim/1 -> Discrete-Time Integrator/1
  Sum4/1 -> Kilim/1, Kplim/1
  Plimit/1 -> Sum4/1
  Kplim1/1 -> Saturation1/1
  Saturation1/1 -> Sum2/1
  Kplim/1 -> Saturation2/1
  Saturation2/1 -> Sum9/1
  Sum9/1 -> Sum3/1
  Sum2/1 -> Sum3/2

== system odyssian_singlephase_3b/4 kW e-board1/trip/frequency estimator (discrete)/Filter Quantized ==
  In : Inport
  Input Quantizer : DataTypeConversion  OutDataTypeMode=Specify via dialog  OutDataType=fixdt(1,16,15)  OutDataTypeStr=fixdt(1,16,15)  RndMeth=Round
  filter : dsparch4/Biquad Filter  DialogController=dspdialog.BiquadFilter  DialogControllerArgs=DataTag0  IIRFiltStruct=Direct form II  CoeffSource=Specify via dialog  BiQuadCoeffs=[1 -1.35890654546667 1 1 -1.77683423091592 0.868775728611993;1 1 0 1 -0.84680556917748 0]  a0Flag=Warning  IC=0  ICnum=0  ICden=0  firstCoeffMode=Binary point scaling  firstCoeffWordLength=16  firstCoeffFracLength=14  outputMode=Binary point scaling  outputWordLength=16  outputFracLength=11  accumMode=Binary point scaling  accumWordLength=40  accumFracLength=29  denAccumFracLength=29  prodOutputMode=Binary point scaling  prodOutputWordLength=32  prodOutputFracLength=29  denProdOutputFracLength=29  memoryMode=Binary point scaling  memoryWordLength=16  memoryFracLength=15  secondMemoryFracLength=15  roundingMode=Convergent  overflowMode=off  ScaleValues=[0.0483208011510974;0.227336456672284;1]  optimizeScaleValues=on  ScaleValueMode=Specify via input port (g)  scaleValueFracLength=17  stageInputMode=Binary point scaling  stageOutputMode=Binary point scaling  stageInputWordLength=16  stageInputFracLength=12  stageOutputWordLength=16  stageOutputFracLength=11  FilterSource=Specify via dialog  dfiltObjectName=dfilt.df2tsos([1 0.3 0.4],[1 0.1 0.2])
  Out : Outport
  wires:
  In/1 -> Input Quantizer/1
  Input Quantizer/1 -> filter/1
  filter/1 -> Out/1

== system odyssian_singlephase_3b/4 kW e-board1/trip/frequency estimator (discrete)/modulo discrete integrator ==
  In1 : Inport
  Abs : Abs
  Constant1 : Constant  OutDataType=sfix(16)  OutScaling=2^0
  Discrete-Time Integrator : DiscreteIntegrator  ExternalReset=rising  InitialConditionSource=external  SampleTime=dt  OutDataType=fixdt(1, 16)  OutScaling=2^0  UpperSaturationLimit=100  LowerSaturationLimit=-100  ShowStatePort=on  ICPrevOutput=DiscIntNeverNeededParam  ICPrevScaledInput=DiscIntNeverNeededParam
  Gain1 : Gain  Gain=1+.0001  ParameterDataType=sfix(16)  ParameterScaling=2^0  OutDataType=sfix(16)  OutScaling=2^0
  IC : InitialCondition  Value=0
  Math Function : Math  Operator=rem  OutDataType=sfix(16)  OutScaling=2^0
  Relational Operator : RelationalOperator
  Out1 : Outport
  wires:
  Relational Operator/1 -> Discrete-Time Integrator/2
  Discrete-Time Integrator/State -> Gain1/1
  Gain1/1 -> Abs/1
  Constant1/1 -> Relational Operator/2, Math Function/2
  Abs/1 -> Relational Operator/1, Math Function/1
  In1/1 -> Discrete-Time Integrator/1
  Discrete-Time Integrator/1 -> Out1/1
  IC/1 -> Discrete-Time Integrator/3
  Math Function/1 -> IC/1

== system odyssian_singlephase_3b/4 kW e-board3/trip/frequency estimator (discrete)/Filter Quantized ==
  In : Inport
  Input Quantizer : DataTypeConversion  OutDataTypeMode=Specify via dialog  OutDataType=fixdt(1,16,15)  OutDataTypeStr=fixdt(1,16,15)  RndMeth=Round
  filter : dsparch4/Biquad Filter  DialogController=dspdialog.BiquadFilter  DialogControllerArgs=DataTag1  IIRFiltStruct=Direct form II  CoeffSource=Specify via dialog  BiQuadCoeffs=[1 -1.35890654546667 1 1 -1.77683423091592 0.868775728611993;1 1 0 1 -0.84680556917748 0]  a0Flag=Warning  IC=0  ICnum=0  ICden=0  firstCoeffMode=Binary point scaling  firstCoeffWordLength=16  firstCoeffFracLength=14  outputMode=Binary point scaling  outputWordLength=16  outputFracLength=11  accumMode=Binary point scaling  accumWordLength=40  accumFracLength=29  denAccumFracLength=29  prodOutputMode=Binary point scaling  prodOutputWordLength=32  prodOutputFracLength=29  denProdOutputFracLength=29  memoryMode=Binary point scaling  memoryWordLength=16  memoryFracLength=15  secondMemoryFracLength=15  roundingMode=Convergent  overflowMode=off  ScaleValues=[0.0483208011510974;0.227336456672284;1]  optimizeScaleValues=on  ScaleValueMode=Specify via input port (g)  scaleValueFracLength=17  stageInputMode=Binary point scaling  stageOutputMode=Binary point scaling  stageInputWordLength=16  stageInputFracLength=12  stageOutputWordLength=16  stageOutputFracLength=11  FilterSource=Specify via dialog  dfiltObjectName=dfilt.df2tsos([1 0.3 0.4],[1 0.1 0.2])
  Out : Outport
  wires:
  In/1 -> Input Quantizer/1
  Input Quantizer/1 -> filter/1
  filter/1 -> Out/1

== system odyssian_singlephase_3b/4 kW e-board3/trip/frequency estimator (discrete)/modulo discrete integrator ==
  In1 : Inport
  Abs : Abs
  Constant1 : Constant  OutDataType=sfix(16)  OutScaling=2^0
  Discrete-Time Integrator : DiscreteIntegrator  ExternalReset=rising  InitialConditionSource=external  SampleTime=dt  OutDataType=fixdt(1, 16)  OutScaling=2^0  UpperSaturationLimit=100  LowerSaturationLimit=-100  ShowStatePort=on  ICPrevOutput=DiscIntNeverNeededParam  ICPrevScaledInput=DiscIntNeverNeededParam
  Gain1 : Gain  Gain=1+.0001  ParameterDataType=sfix(16)  ParameterScaling=2^0  OutDataType=sfix(16)  OutScaling=2^0
  IC : InitialCondition  Value=0
  Math Function : Math  Operator=rem  OutDataType=sfix(16)  OutScaling=2^0
  Relational Operator : RelationalOperator
  Out1 : Outport
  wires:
  Relational Operator/1 -> Discrete-Time Integrator/2
  Discrete-Time Integrator/State -> Gain1/1
  Gain1/1 -> Abs/1
  Constant1/1 -> Relational Operator/2, Math Function/2
  Abs/1 -> Relational Operator/1, Math Function/1
  In1/1 -> Discrete-Time Integrator/1
  Discrete-Time Integrator/1 -> Out1/1
  IC/1 -> Discrete-Time Integrator/3
  Math Function/1 -> IC/1
